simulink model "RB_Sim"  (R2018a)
settings: Solver=ode45  StartTime=0.0  StopTime=25  RelTol=1e-3  EnableMultiTasking=on
InitFcn:
  | init
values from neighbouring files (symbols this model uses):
  d2r = pi/180    (= 0.0174532925199)    [init.m]    (also in LQR_Design.m)
  r2d = 1/d2r    (= 57.2957795131)    [init.m]    (also in LQR_Design.m)
undefined symbols (not defined in the file or in its folder): Av, Bv, Cv, Dv, Kmix, Kpr, Kq

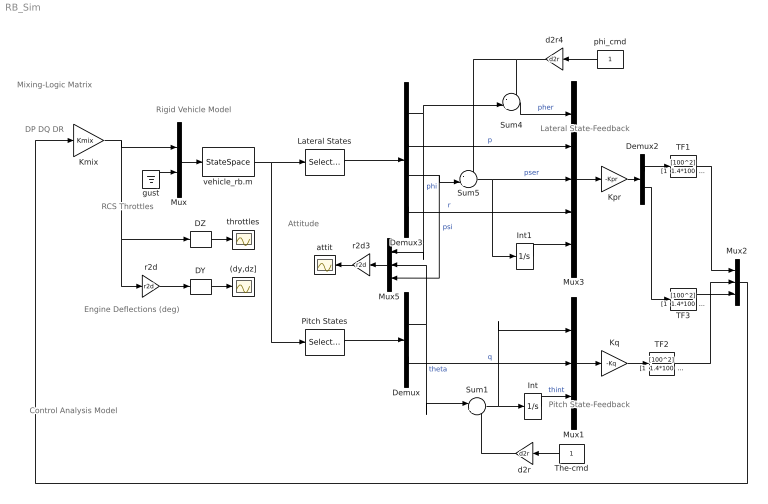
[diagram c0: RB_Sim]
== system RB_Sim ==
  note: Control Analysis Model
  note: Rigid Vehicle Model
  note: Pitch State-Feedback
  note: Lateral State-Feedback
  note: Mixing-Logic Matrix
  note: Engine Deflections (deg)
  note: RCS Throttles
  note: DP DQ DR
  note: Attitude
  (dy,dz] : Scope
  DY : Selector  InputPortWidth=6  IndexOptions=Index vector (dialog)  Indices=[1,2]  OutputSizes=1
  DZ : Selector  InputPortWidth=6  IndexOptions=Index vector (dialog)  Indices=[3:6]  OutputSizes=1
  Demux : Demux  Outputs=2
  Demux2 : Demux  Outputs=2
  Demux3 : Demux
  Int : Integrator
  Int1 : Integrator
  Kmix : Gain  Gain=Kmix  Multiplication=Matrix(K*u)
  Kpr : Gain  Gain=-Kpr  Multiplication=Matrix(K*u)
  Kq : Gain  Gain=-Kq  Multiplication=Matrix(K*u)
  Lateral States : Selector  InputPortWidth=14  IndexOptions=Index vector (dialog)  Indices=[1,2, 5,6]  OutputSizes=1
  Mux : Mux  Inputs=[6,1]
  Mux1 : Mux  Inputs=3
  Mux2 : Mux  Inputs=3
  Mux3 : Mux  Inputs=5
  Mux5 : Mux  Inputs=3
  Pitch States : Selector  InputPortWidth=14  IndexOptions=Index vector (dialog)  Indices=[3, 4]  OutputSizes=1
  Sum1 : Sum  Inputs=|+-
  Sum4 : Sum  Inputs=-+|
  Sum5 : Sum  Inputs=-+|
  TF1 : TransferFcn  Numerator=[100^2]  Denominator="[1  1.4*100  100^2]"
  TF2 : TransferFcn  Numerator=[100^2]  Denominator="[1  1.4*100  100^2]"
  TF3 : TransferFcn  Numerator=[100^2]  Denominator="[1  1.4*100  100^2]"
  The-cmd : Constant
  attit : Scope
  d2r : Gain  Gain=d2r
  d2r4 : Gain  Gain=d2r
  gust : Ground
  phi_cmd : Constant
  r2d : Gain  Gain=r2d
  r2d3 : Gain  Gain=r2d
  throttles : Scope
  vehicle_rb.m : StateSpace  A=Av  B=Bv  C=Cv  D=Dv  InitialCondition=0
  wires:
  Mux/1 -> vehicle_rb.m/1
  Kmix/1 -> r2d/1, DZ/1, Mux/1
  gust/1 -> Mux/2
  vehicle_rb.m/1 -> Pitch States/1, Lateral States/1
  Demux/2 -> Mux1/2  "q"
  Pitch States/1 -> Demux/1
  Mux1/1 -> Kq/1
  Demux/1 -> Mux5/2, Sum1/1  "theta"
  Kq/1 -> TF2/1
  The-cmd/1 -> d2r/1
  Demux3/2 -> Mux3/2  "p"
  Demux3/4 -> Mux3/4  "r"
  Demux3/3 -> Mux5/3, Sum5/2  "psi"
  Sum5/1 -> Mux3/3, Int1/1  "pser"
  Kpr/1 -> Demux2/1
  Demux2/1 -> TF1/1
  Demux2/2 -> TF3/1
  Sum4/1 -> Mux3/1  "pher"
  Demux3/1 -> Mux5/1, Sum4/2  "phi"
  phi_cmd/1 -> d2r4/1
  Mux2/1 -> Kmix/1
  DZ/1 -> throttles/1
  DY/1 -> (dy,dz]/1
  d2r4/1 -> Sum5/1, Sum4/1
  r2d/1 -> DY/1
  Lateral States/1 -> Demux3/1
  Mux3/1 -> Kpr/1
  Int1/1 -> Mux3/5
  Sum1/1 -> Mux1/1, Int/1
  d2r/1 -> Sum1/2
  Int/1 -> Mux1/3  "thint"
  Mux5/1 -> r2d3/1
  r2d3/1 -> attit/1
  TF2/1 -> Mux2/2
  TF1/1 -> Mux2/1
  TF3/1 -> Mux2/3
